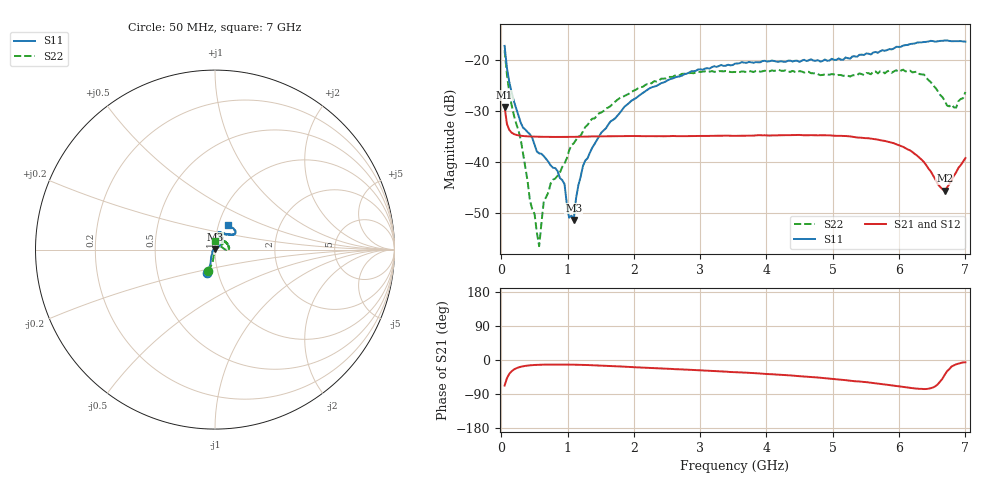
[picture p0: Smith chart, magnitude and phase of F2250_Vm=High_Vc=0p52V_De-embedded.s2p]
! Integrated Device Technology
! Corporate Headquarters
! 6024 Silver Creek Valley Road
! San Jose, CA 95138  USA
! Phone:  1-408-284-8200
! Toll Free:  1-800-223-1366
! Webpage:  http://www.idt.com/
! Timing and RF Division
! 515 Groton Road, Suite 102
! Westford, MA 01886-6024
! Device:  F2250
! Description: Voltage Variable RF Attenuator
! Frequency:  50.0 -  6000.00 MHz
! Package:  3x3 mm Thin QFN Plastic Package: 16 pin
! Ports:  2 RF, 3 DC
!  Pin  1  = GND
!  Pin  2  = NC
!  Pin  3  = RF1  = Port 1
!  Pin  4  = NC
!  Pin  5  = GND
!  Pin  6  = GND
!  Pin  7  = GND
!  Pin  8  = GND
!  Pin  9  = NC
!  Pin 10  = RF2  = Port 2
!  Pin 11  = NC
!  Pin 12  = GND
!  Pin 13  = GND
!  Pin 14  = VCNTRL
!  Pin 15  = VDD
!  Pin 16  = VMODE
! Vcntrl:  0.520 Volts
! Vmode:  +3.300 Volts
! Vdd:  +3.30  Volts
! Current:  1.271 mA
! Data:  The device was measured on a the F2250 evaluation board which has
!  individual transmission lines to the RF pins.  Data was collected
!  using a calibrated network analyzer.  The evaluation board was
!  de-embedded using a TRL calibration technique.
!  The reference plane is the edge of the package pin.
! Misc:  SN 10
!  Action Tracker AT0258
! Date Measured:  2014-11-26
! Date:  2015-10-15  MJV
! Note:
!  Integrated Device Technology supplies this data as a sample of measured
!  data at the package pin for this product.  Your particular data for this
!  product may vary.
!  Data was taken at 25 degrees C.
!  Integrated Device Technology reserves the right to change this data at anytime.
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# GHz S dB R 50
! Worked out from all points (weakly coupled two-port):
!   201 points, 50 MHz to 7 GHz, reference 50 ohm
!   highest |S21| = -29.19 dB at 50 MHz (marker M1); lowest = -45.7 dB at 6.687 GHz (marker M2)
!   lowest |S11| = -51.4 dB at 1.093 GHz (marker M3), VSWR 1.01, Z = 50 + j0.269 ohm
!   |S11| at or under -10 dB: start of sweep to end of sweep
!   |S22| runs from -56.6 to -18.0 dB; largest |S21 - S12| = 5.5e-05
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0.05  -17.17 -108.4  -29.19 -67.4  -29.19 -67.4  -18.04 -107.1
0.08475  -21.47 -107.3  -32.51 -48.3  -32.51 -48.3  -22.78 -100.4
0.15425  -26.22 -116.4  -34.22 -29.8  -34.22 -29.8  -28.74 -102.9
0.29325  -32.28 -127.1  -34.85 -17.9  -34.85 -17.9  -35.57 -94.7
0.43225  -34.56 -145.1  -34.99 -14.0  -34.99 -14.1  -47.64 -88.3
0.50175  -36.65 -147.5  -35.02 -13.1  -35.02 -13.2  -50.23 -81.7
0.57125  -38.31 -160.9  -35.04 -12.6  -35.05 -12.6  -56.57 -27.6
0.64075  -38.85 -162.2  -35.06 -12.2  -35.07 -12.2  -47.77 22.3
0.9535  -44.36 170.8  -35.09 -12.1  -35.09 -12.1  -40.31 44.9
1.023  -50.98 140.2  -35.08 -12.2  -35.08 -12.2  -37.76 39.6
1.0925  -51.41 87.9  -35.07 -12.4  -35.07 -12.4  -36.34 39.7
1.12725  -47.17 60.3  -35.05 -12.5  -35.06 -12.6  -35.65 35.8
1.2315  -40.82 40.2  -35.02 -12.9  -35.03 -13.0  -34.02 31.1
1.6485  -32.02 40.9  -34.95 -15.8  -34.95 -15.8  -29.01 36.0
2.37825  -24.75 46.5  -34.93 -21.9  -34.93 -21.9  -24.00 40.8
3.525  -20.66 71.7  -34.87 -31.9  -34.87 -32.0  -22.30 65.6
4.7065  -20.07 72.0  -34.74 -45.4  -34.74 -45.4  -22.57 65.9
5.85325  -17.80 40.5  -36.11 -66.1  -36.12 -66.2  -22.05 16.4
6.3745  -16.40 40.9  -40.02 -76.7  -40.04 -76.7  -22.80 -0.1
6.68725  -16.12 47.8  -45.66 -39.4  -45.65 -39.0  -27.90 22.0
6.861  -16.22 54.5  -42.04 -11.3  -42.01 -11.3  -29.31 58.9
7  -16.33 62.4  -39.24 -6.1  -39.21 -6.3  -26.24 89.8
